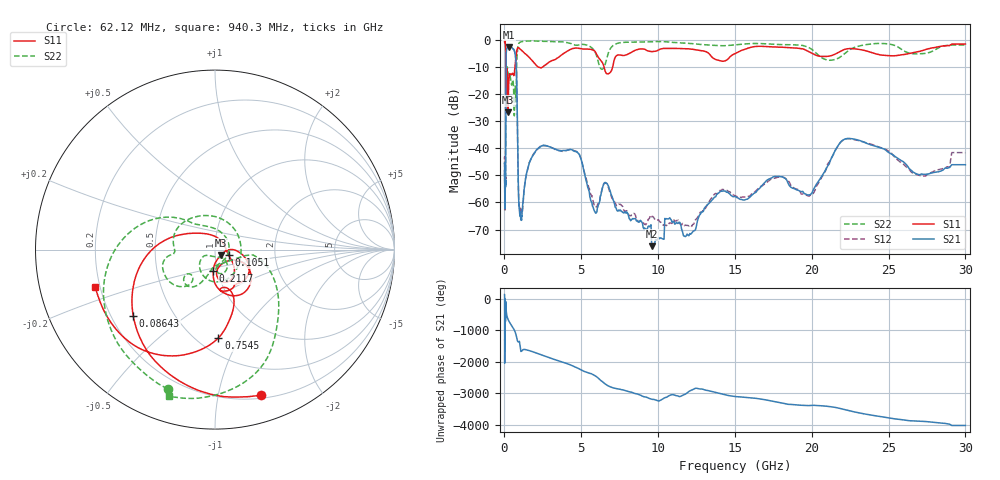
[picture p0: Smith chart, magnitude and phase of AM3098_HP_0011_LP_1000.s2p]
! Date/Time: Thu, Feb 28, 2019 8:34 AM
! Network Analyzer: Agilent Technologies E8364B Rev: A.07.50.67
! Sweep from 0.010 to 30.000 GHz, 1601 Points, Sweep Type: LOG
! Power Supply: 5.022 V, 0.002 A
# Hz S DB R 50
!freq MagS11 AngS11 MagS21 AngS21 MagS12 AngS12 MagS22 AngS22
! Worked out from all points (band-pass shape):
!   1601 points, 10 MHz to 30 GHz, reference 50 ohm
!   highest |S21| = -2.74 dB at 271.8 MHz (marker M1); lowest = -76.1 dB at 9.586 GHz (marker M2)
!   |S21| within 3 dB of the highest: 108.6 MHz to 706.2 MHz (597.6 MHz wide, 147 % of centre)
!   lowest |S11| = -26.8 dB at 235.1 MHz (marker M3), VSWR 1.10, Z = 53.3 - j3.37 ohm
!   |S11| at or under -10 dB: 93.02 MHz to 682.4 MHz (589.4 MHz wide, 152 % of centre); 2.161 GHz to 2.516 GHz (355.1 MHz wide, 15.2 % of centre); 6.479 GHz to 7.048 GHz (569 MHz wide, 8.41 % of centre)
!   |S22| runs from -28.1 to -0.5 dB; largest |S21 - S12| = 0.011
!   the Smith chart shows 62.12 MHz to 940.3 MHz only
!   S11 on the Smith chart (normalised r, x): 62.12 MHz: 0.23, -1.34; 86.43 MHz: 0.29, -0.33; 105.1 MHz: 1.16, -0.07; 211.7 MHz: 0.95, -0.23; 754.5 MHz: 0.63, -0.82; 940.3 MHz: 0.18, -0.15
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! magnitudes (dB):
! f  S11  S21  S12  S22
! 10 MHz  -0.4  -45.8  -44.4  -0.6
! 38.04 MHz  -0.5  -59.3  -60.6  -0.9
! 62.12 MHz  -1.4  -52.0  -51.9  -1.7
! 75.13 MHz  -2.2  -53.6  -50.9  -2.6
! 86.43 MHz  -4.6  -29.9  -29.9  -5.1
! 105.1 MHz  -21.7  -6.5  -6.5  -15.3
! 144.7 MHz  -15.7  -3.5  -3.4  -13.1
! 211.7 MHz  -18.3  -3.0  -2.9  -11.7
! 235.1 MHz  -26.8  -2.8  -2.8  -12.6
! 271.8 MHz  -17.0  -2.7  -2.7  -12.9
! 550.5 MHz  -12.7  -3.4  -3.4  -14.9
! 639.6 MHz  -12.7  -4.1  -4.0  -28.1
! 754.5 MHz  -6.2  -8.7  -8.7  -19.4
! 940.3 MHz  -3.1  -61.1  -59.8  -1.3
! 2.084 GHz  -9.6  -40.6  -40.7  -0.6
! 4.687 GHz  -3.1  -41.3  -41.2  -2.1
! 5.812 GHz  -4.0  -62.5  -60.4  -3.8
! 7.926 GHz  -5.7  -63.9  -63.0  -1.0
! 9.586 GHz  -4.5  -76.1  -65.2  -0.9
! 19.7 GHz  -4.2  -57.2  -57.5  -2.7
! 22.56 GHz  -3.3  -36.5  -36.6  -3.5
! 30 GHz  -1.7  -46.1  -41.6  -2.0
